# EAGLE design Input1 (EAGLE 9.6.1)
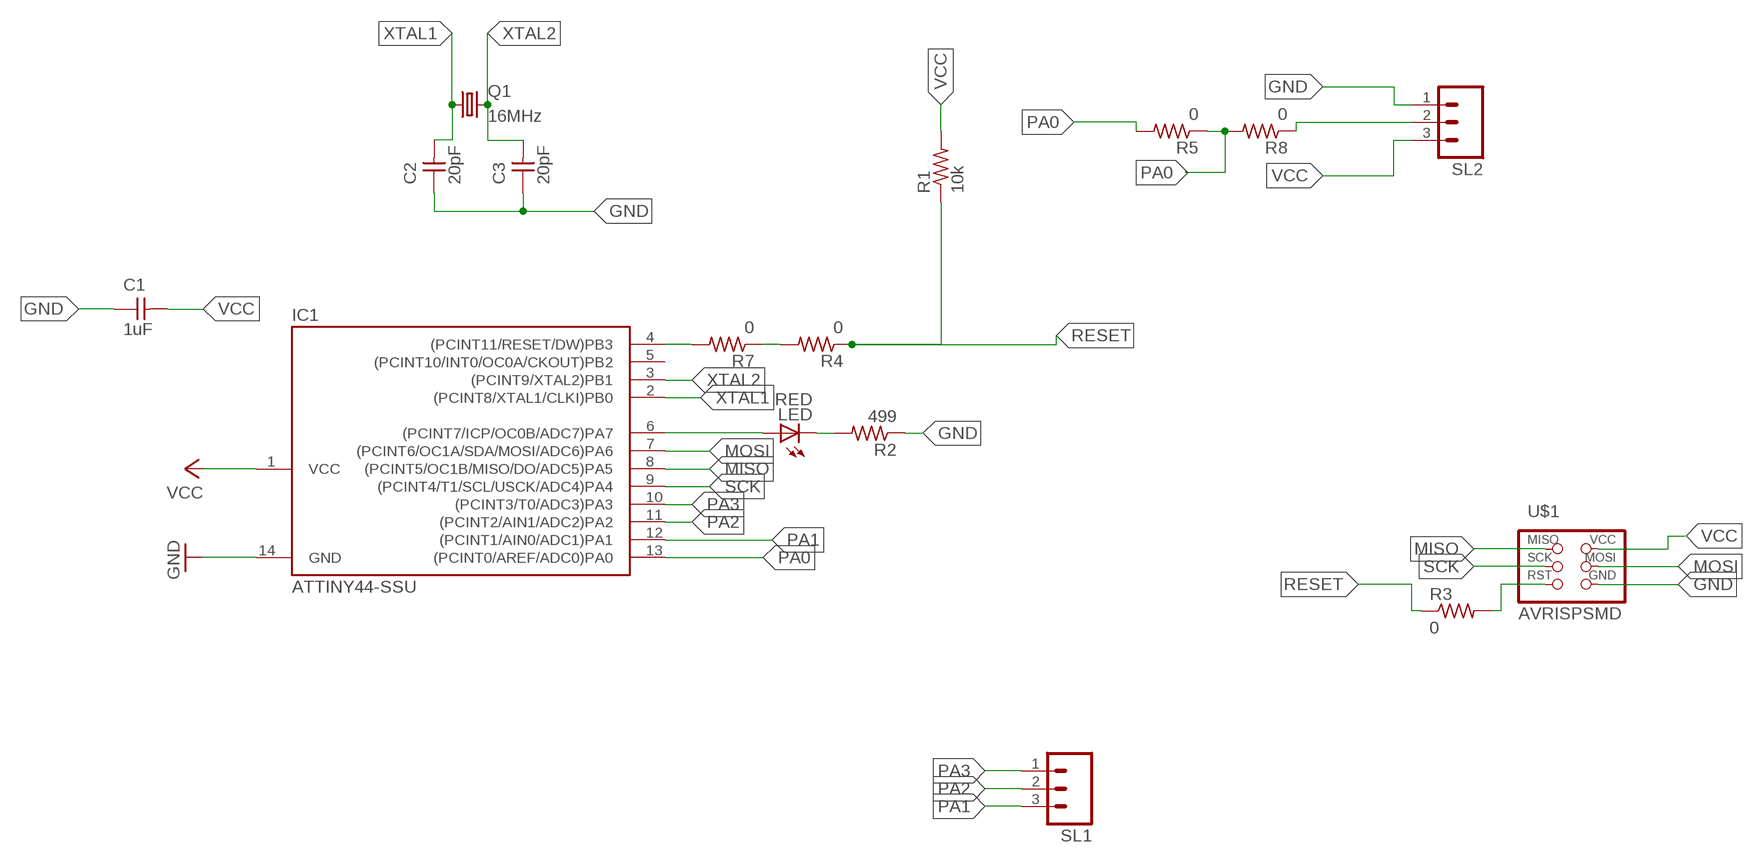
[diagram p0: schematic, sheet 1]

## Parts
C1  1uF  UNPOLARIZED_CAPACITOR1206  [1206]
C2  20pF  UNPOLARIZED_CAPACITOR1206  [1206]
C3  20pF  UNPOLARIZED_CAPACITOR1206  [1206]
IC1  ATTINY44-SSU  [SOIC14]
LED  RED  LED1206  [1206]
Q1  16MHz  CSM-7X-DU  [CSM-7X-DU]
R1  10k  RES-US1206  [R1206]
R2  499  RESISTOR1206  [1206]
R3  0  RES-US1206  [R1206]
R4  0  RES-US1206  [R1206]
R5  0  RES-US1206  [R1206]
R7  0  RES-US1206  [R1206]
R8  0  RES-US1206  [R1206]
SL1  M03  [03P]
SL2  M03  [03P]
U$1  AVRISPSMD  [2X03SMD]

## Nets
GND: C1.1 C2.1 C3.1 IC1.14(GND) R2.1 SL2.1 U$1.6(GND)
MISO: IC1.8((PCINT5/OC1B/MISO/DO/ADC5)PA5) U$1.1(MISO)
MOSI: IC1.7((PCINT6/OC1A/SDA/MOSI/ADC6)PA6) U$1.4(MOSI)
N$1: IC1.6((PCINT7/ICP/OC0B/ADC7)PA7) LED.1(A)
N$2: LED.2(C) R2.2
N$3: R3.2 U$1.5(RST)
N$4: R4.2 R7.1
N$6: IC1.4((PCINT11/RESET/DW)PB3) R7.2
N$7: R8.1 SL2.2
PA0: IC1.13((PCINT0/AREF/ADC0)PA0) R5.1 R5.2 R8.2
PA1: IC1.12((PCINT1/AIN0/ADC1)PA1) SL1.3
PA2: IC1.11((PCINT2/AIN1/ADC2)PA2) SL1.2
PA3: IC1.10((PCINT3/T0/ADC3)PA3) SL1.1
RESET: R1.1 R3.1 R4.1
SCK: IC1.9((PCINT4/T1/SCL/USCK/ADC4)PA4) U$1.3(SCK)
VCC: C1.2 IC1.1(VCC) R1.2 SL2.3 U$1.2(VCC)
XTAL1: C2.2 IC1.2((PCINT8/XTAL1/CLKI)PB0) Q1.1
XTAL2: C3.2 IC1.3((PCINT9/XTAL2)PB1) Q1.2
Unconnected: IC1.5((PCINT10/INT0/OC0A/CKOUT)PB2)

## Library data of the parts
C1-C3 = FAB_Hello:UNPOLARIZED_CAPACITOR: unpolarized_capacitor
IC1 = FAB_Hello:ATTINY44
LED = FAB_Hello:LED
Q1 = FAB_Hello:CSM-7X-DU: SMD CRYSTAL; OC_FARNELL: unknown; OC_NEWARK: unknown
R1 R3-R5 R7 R8 = fab:RES-US: Resistor (US Symbol)
R2 = FAB_Hello:RESISTOR
SL1 SL2 = con-amp-quick:M03: AMP QUICK CONNECTOR; OC_FARNELL: unknown; OC_NEWARK: unknown
U$1 = FAB_Hello:AVRISP

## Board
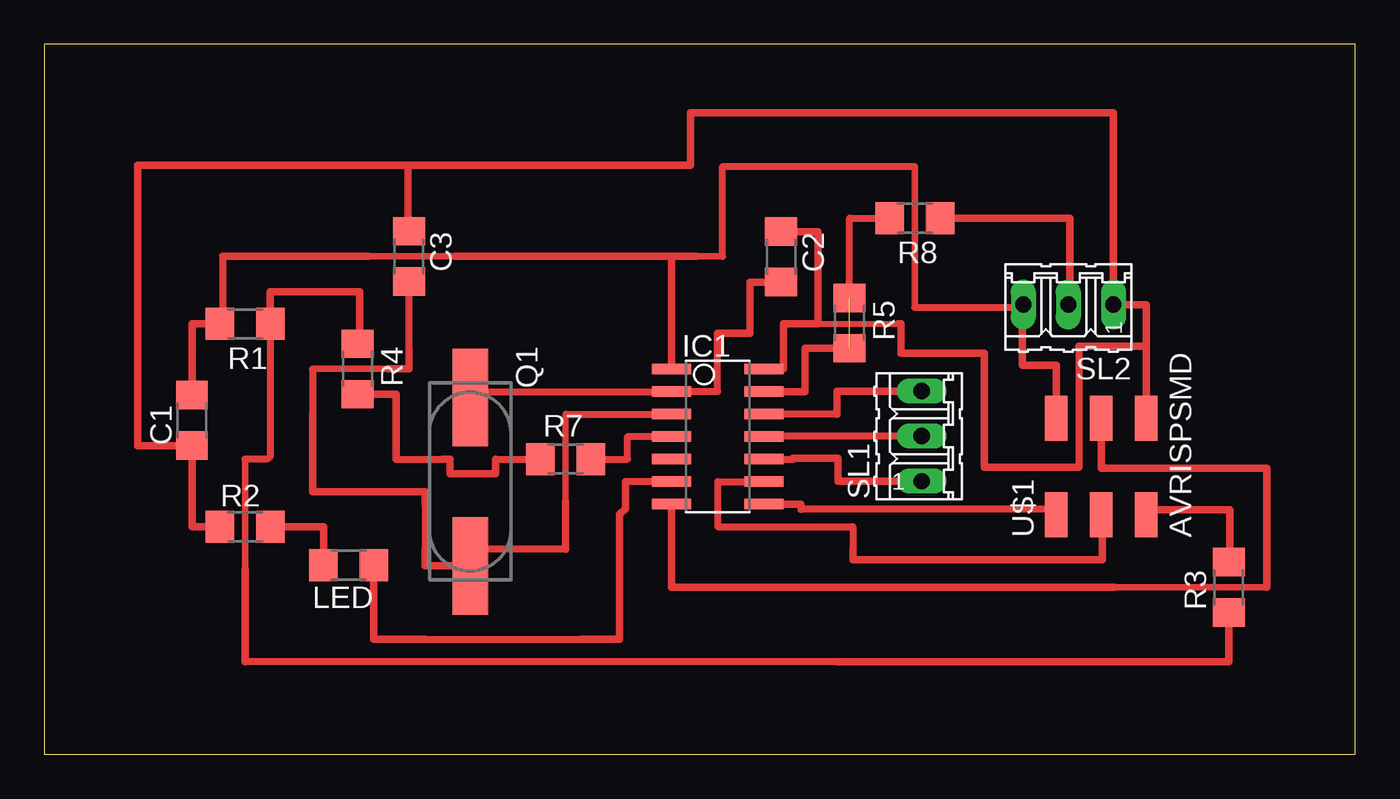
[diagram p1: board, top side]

Size 73.97 x 40.06 mm. Coordinates in mm from the lower left corner, seen from the top.
Outline: 0,0 73.97,0 73.97,40.06 0,40.06 0,0
Copper layers (1*16): Top 0.035mm / dielectric 1.5mm / Bottom 0.035mm
Design rules "default *": minimum track width 6mil, minimum drill 0.35mm, track to track 17mil, track to pad 17mil, pad to pad 17mil, via to via 17mil, smd to smd 17mil, copper to edge 40mil, drill to drill 6mil, minimum pad ring 10mil, minimum via ring 8mil, stop-mask expansion 4mil, vias tented up to drill 0mil, thermal gap 17mil

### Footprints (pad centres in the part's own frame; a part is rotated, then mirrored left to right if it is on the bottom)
1206 = smd 1.6 x 1.803: 1 -1.422,0; 2 1.422,0
SOIC14 = smd 0.61 x 2.21: 1 -3.81,-2.603; 2 -2.54,-2.603; 3 -1.27,-2.603; 4 0,-2.603; 5 1.27,-2.603; 6 2.54,-2.603; 7 3.81,-2.603; 8 3.81,2.603; 9 2.54,2.603; 10 1.27,2.603; 11 0,2.603; 12 -1.27,2.603; 13 -2.54,2.603; 14 -3.81,2.603
CSM-7X-DU = smd 5.5 x 2: 1 -4.75,0; 2 4.75,0
R1206 = smd 1.6 x 1.803: 1 -1.422,0; 2 1.422,0
03P = drill 0.914 long: 1 -2.54,0; 2 0,0; 3 2.54,0
2X03SMD = smd 2.54 x 1.27: 1 -2.54,2.54; 2 2.92,2.54; 3 -2.54,0; 4 2.92,0; 5 -2.54,-2.54; 6 2.92,-2.54

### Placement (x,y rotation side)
C1  8.33,18.85 90 top
C2  41.58,28.07 270 top
C3  20.57,28.09 270 top
IC1  38,17.93 270 top
LED  17.17,10.67 180 top
Q1  24.03,15.39 270 top
R1  11.33,24.28 180 top
R2  11.33,12.85 0 top
R3  66.83,9.42 90 top
R4  17.68,21.74 270 top
R5  45.44,24.33 270 top
R7  29.41,16.66 0 top
R8  49.12,30.25 180 top
SL1  49.5,17.96 90 top
SL2  57.79,25.37 180 top
U$1  59.64,16.05 90 top

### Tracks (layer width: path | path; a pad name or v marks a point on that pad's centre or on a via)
GND
  Top 0.33: 43.66,24.31 48.18,24.31
  Top 0.381: 58.37,23.01 58.37,16.21
  Top 0.432: 20.52,33.25 36.47,33.25 36.47,36.2 60.33,36.2 SL2.1 62.18,25.37 62.18,23.01 | C2.1 43.66,29.49 43.66,24.31 41.72,24.31 41.72,21.74 IC1.14 | C3.1 20.52,29.51 20.52,33.25 | 48.18,24.31 48.34,24.31 48.34,22.63 53.06,22.63 53.06,16.21 58.37,16.21 | 62.18,23.01 U$1.6 | 62.18,23.01 58.37,23.01 | R2.1 8.33,12.85 C1.1 5.28,17.42 5.28,33.25 20.52,33.25
MISO
  Top 0.406: 42.7,13.84 56.77,13.84 U$1.1
  Top 0.432: IC1.8 42.7,14.12 42.7,13.84
MOSI
  Top 0.356: 68.99,9.42 60.38,9.42
  Top 0.432: U$1.4 59.64,16.15 68.99,16.15 68.99,9.42 | 60.38,9.42 35.39,9.42 IC1.7
N$1
  Top 0.406: 21.49,6.5 30.28,6.5 | IC1.6 32.89,15.39
  Top 0.432: 21.49,6.5 18.59,6.5 LED.1 | 30.28,6.5 32.46,6.5 32.46,13.54 32.79,13.87 32.79,15.39 32.89,15.39
N$2
  Top 0.432: R2.2 15.75,12.85 LED.2
N$3
  Top 0.432: U$1.5 62.18,13.79 66.9,13.79 66.9,10.85 R3.2
N$4
  Top 0.406: 19.84,16.66 22.45,16.66 | 25.45,16.66 R7.1
  Top 0.432: R4.2 19.84,20.32 19.84,16.66 | 22.45,16.66 22.89,16.66 22.89,15.82 25.45,15.82 25.45,16.66
N$6
  Top 0.406: IC1.4 32.92,17.93 32.92,16.66 R7.2
N$7
  Top 0.432: SL2.2 57.86,25.45 57.86,30.25 R8.1
PA0  (1 unrouted)
  Top 0.406: R5.1 45.44,30.25 R8.2
  Top 0.432: IC1.13 42.93,20.47 42.93,22.91 R5.2
PA1
  Top 0.406: 44.73,19.2 IC1.12
  Top 0.432: SL1.3 44.73,20.5 44.73,19.2
PA2
  Top 0.406: IC1.11 40.63,17.96 SL1.2
PA3
  Top 0.406: IC1.10 42.24,16.66
  Top 0.432: SL1.1 44.78,15.42 44.78,16.71 42.24,16.71 42.24,16.66
RESET
  Top 0.356: 11.33,16.66 11.33,10.46
  Top 0.406: R1.1 12.75,16.81 12.6,16.66 11.33,16.66 | 44.73,5.23 11.33,5.23
  Top 0.432: 11.33,10.46 11.33,5.23 | R3.1 66.83,5.23 44.73,5.23 | R1.1 12.75,26.09 17.78,26.09 17.78,23.16 R4.1
SCK
  Top 0.406: IC1.9 38,15.39 38,12.85 45.62,12.85 45.62,11.58
  Top 0.432: 45.62,11.58 45.62,10.97 59.72,10.97 59.72,13.51 U$1.3
VCC
  Top 0.356: 49.12,33.17 49.12,25.2 | 38.28,28.09 36.8,28.09 | 23.19,28.09 18.29,28.09
  Top 0.406: 49.12,33.17 38.28,33.17 38.28,28.09 | R1.2 10.06,24.43 10.06,28.09 | SL2.3 55.07,25.2 49.12,25.2
  Top 0.432: U$1.2 57.1,21.95 55.19,21.95 55.19,25.37 SL2.3 | R1.2 8.33,24.28 C1.2 | 23.19,28.09 35.28,28.09 35.39,28.09 | 35.39,28.09 36.8,28.09 | 18.29,28.09 10.06,28.09 | IC1.1 35.39,28.09
XTAL1
  Top 0.406: Q1.1 24.36,20.47 IC1.2 38,20.47 38,22.66
  Top 0.432: 38,22.66 38,23.75 39.83,23.75 39.83,26.65 C2.2
XTAL2
  Top 0.356: 29.41,19.2 29.41,14.27 | 15.14,21.74 19.41,21.74
  Top 0.406: Q1.2 24.97,11.58 29.41,11.58 | 29.41,19.2 IC1.3 | 15.14,21.74 15.14,19.2 | 21.49,14.12 21.49,11.58 | 20.57,22.89 C3.2
  Top 0.432: Q1.2 21.49,10.64 21.49,11.58 | 21.49,14.12 21.49,14.81 15.14,14.81 15.14,19.2 | 19.41,21.74 20.57,21.74 20.57,22.89 | 29.41,14.27 29.41,11.58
